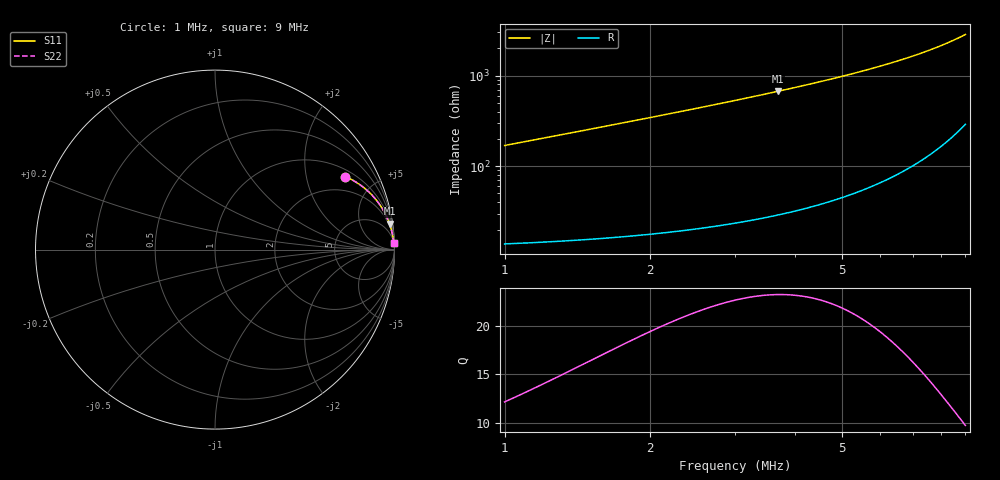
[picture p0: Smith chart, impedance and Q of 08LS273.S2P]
! Coilcraft 0805LS-273 Chip Inductor
! 18 September 2002
# MHZ S MA R 50
!Freq  MagS11  AngS11  MagS21  AngS21  MagS12  AngS12  MagS22  AngS22
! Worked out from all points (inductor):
!   401 points, 1 MHz to 9 MHz, reference 50 ohm
!   read as one part in series: L = 27.1 uH near 1.04 MHz
!   highest Q = 23.2 at 3.68 MHz (marker M1), where L = 29 uH
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1  0.8317 29.3  0.4913 -56.0  0.4913 -56.0  0.8317 29.3
1.04  0.8414 28.4  0.4777 -57.0  0.4777 -57.0  0.8414 28.4
1.16  0.8661 26.1  0.4405 -59.7  0.4405 -59.7  0.8661 26.1
1.28  0.8858 24.0  0.4077 -62.1  0.4077 -62.1  0.8858 24.0
1.42  0.9039 21.9  0.3743 -64.4  0.3743 -64.4  0.9039 21.9
1.56  0.9182 20.2  0.3453 -66.4  0.3453 -66.4  0.9182 20.2
1.72  0.931 18.4  0.3167 -68.4  0.3167 -68.4  0.931 18.4
1.9  0.9421 16.8  0.289 -70.2  0.289 -70.2  0.9421 16.8
2.1  0.9517 15.2  0.2629 -71.9  0.2629 -71.9  0.9517 15.2
2.34  0.9603 13.7  0.2366 -73.6  0.2366 -73.6  0.9603 13.7
2.64  0.9682 12.1  0.2096 -75.3  0.2096 -75.3  0.9682 12.1
2.96  0.9743 10.7  0.1861 -76.7  0.1861 -76.7  0.9743 10.7
3.3  0.979 9.5  0.1656 -78.0  0.1656 -78.0  0.979 9.5
3.68  0.9829 8.4  0.1466 -79.1  0.1466 -79.1  0.9829 8.4
4.28  0.9871 7.0  0.1228 -80.5  0.1228 -80.5  0.9871 7.0
5  0.9903 5.8  0.1009 -81.6  0.1009 -81.6  0.9903 5.8
5.64  0.9922 4.9  0.08545 -82.3  0.08545 -82.3  0.9922 4.9
6.34  0.9935 4.1  0.07159 -82.8  0.07159 -82.8  0.9935 4.1
7.68  0.9951 2.9  0.05079 -83.0  0.05079 -83.0  0.9951 2.9
8.3  0.9955 2.5  0.04293 -82.8  0.04293 -82.8  0.9955 2.5
8.96  0.9958 2.0  0.03544 -82.2  0.03544 -82.2  0.9958 2.0
9  0.9958 2.0  0.03501 -82.2  0.03501 -82.2  0.9958 2.0
